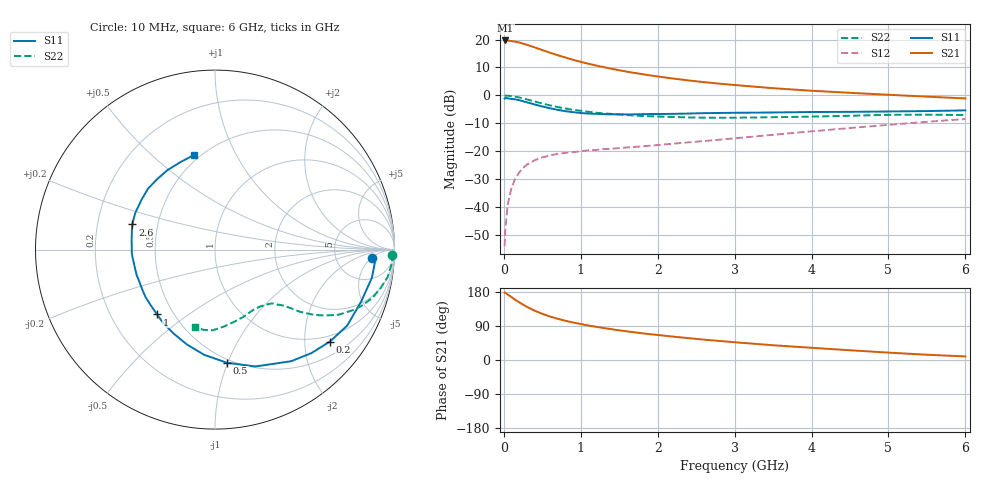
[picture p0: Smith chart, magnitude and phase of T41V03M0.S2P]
! Infineon Technologies  Discrete & RF Semiconductors
! BFR182T
! Si NPN RF Bipolar Junction Transistor in SC75
! VCE = 1 V  IC = 3 mA
! Common Emitter S-Parameters:  October  1999
# GHz  S  MA  R  50
!  f  S11  S21  S12  S22
! GHz  MAG  ANG  MAG  ANG  MAG  ANG  MAG  ANG
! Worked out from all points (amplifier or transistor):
!   36 points, 10 MHz to 6 GHz, reference 50 ohm
!   highest |S21| = 19.7 dB at 20 MHz (marker M1)
!   |S21| within 3 dB of that: start of sweep to 454.4 MHz
!   unconditionally stable (mu >= 1): 1.604 GHz to 4.525 GHz
!   at 250 MHz: K = 0.20, MSG = 22.3 dB, |S12| = -26.0 dB
!   at 1.4 GHz: K = 0.93, MSG = 14.3 dB, |S12| = -19.1 dB
!   at 6 GHz: K = 0.89, MSG = 3.7 dB, |S12| = -8.4 dB
!   S11 on the Smith chart (normalised r, x): 10 MHz: 13, -5; 200 MHz: 0.84, -2.61; 500 MHz: 0.47, -0.99; 1 GHz: 0.41, -0.38; 2.6 GHz: 0.36, +0.13; 6 GHz: 0.46, +0.69
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0.01  0.8787 -3.1  9.561 178.0  0.002 86.0  0.9852 -1.6
0.02  0.897 -2.8  9.639 177.4  0.0041 96.1  0.9917 -1.8
0.05  0.8882 -10.2  9.576 172.7  0.011 87.1  0.9878 -4.6
0.1  0.8642 -19.6  9.382 166.0  0.0222 80.6  0.9744 -9.0
0.15  0.8496 -29.9  9.163 158.7  0.0328 74.2  0.9471 -13.1
0.2  0.8199 -38.7  8.858 152.2  0.042 70.8  0.9191 -16.8
0.25  0.7877 -47.1  8.449 146.1  0.0501 65.6  0.8838 -20.2
0.3  0.7528 -55.7  8.057 140.3  0.0577 62.1  0.8499 -23.1
0.4  0.6891 -70.9  7.25 130.1  0.0692 55.6  0.7779 -27.8
0.5  0.6341 -84.0  6.486 121.9  0.0777 51.3  0.7171 -30.8
0.6  0.5888 -96.0  5.815 114.7  0.0844 48.6  0.6635 -33.3
0.7  0.5514 -106.5  5.251 108.8  0.0898 46.2  0.6191 -34.9
0.8  0.5218 -116.0  4.772 103.5  0.0934 44.5  0.5827 -36.3
1  0.4844 -131.8  3.987 94.9  0.1 43.5  0.5311 -37.7
1.1  0.4731 -139.8  3.692 90.9  0.1038 43.4  0.5089 -38.8
1.5  0.4589 -161.9  2.822 78.3  0.1138 44.5  0.4555 -41.9
2.2  0.4679 173.2  2.006 61.7  0.1366 49.1  0.4112 -49.3
2.6  0.4814 163.1  1.731 53.8  0.1524 51.6  0.3999 -54.7
3.5  0.4949 145.7  1.346 38.9  0.197 54.9  0.4075 -67.9
4.5  0.5078 129.5  1.113 25.7  0.2609 54.4  0.4322 -83.7
5.5  0.5245 111.3  0.95 13.9  0.3372 50.5  0.4516 -98.1
6  0.5398 102.6  0.884 9.4  0.3783 47.2  0.4463 -104.7
